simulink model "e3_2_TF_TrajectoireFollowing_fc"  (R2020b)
settings: Solver=FixedStepAuto  StartTime=0.0  StopTime=100  FixedStep=sampleTime  RelTol=1e-3  EnableMultiTasking=on
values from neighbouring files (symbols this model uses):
  saturation_psi = 2    [startSimulation.m]    (also in StartSimulation.m; start.m)
  saturation_x = 2    [startSimulation.m]    (also in StartSimulation.m; start.m)
  saturation_y = 2    [startSimulation.m]    (also in StartSimulation.m; start.m)
  saturation_z = 2    [startSimulation.m]    (also in StartSimulation.m; start.m)
libraries: simulink x11, aerolibanimutils x1

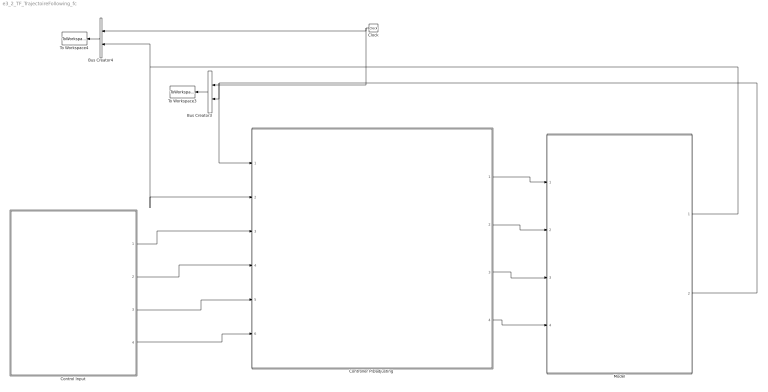
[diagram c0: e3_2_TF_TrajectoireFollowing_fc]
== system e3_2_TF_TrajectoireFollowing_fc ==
  Bus Creator3 : BusCreator  Inputs=2
  Bus Creator4 : BusCreator  Inputs=2
  Clock : Clock
  Control Input : Subsystem
  "Controller PIDadjusting " : Subsystem
  Model : Subsystem
  To Workspace3 : ToWorkspace  VariableName=r1_pos_array  SampleTime=-1
  To Workspace4 : ToWorkspace  VariableName=r1_vel_array  SampleTime=-1
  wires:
  Clock/1 -> Bus Creator4/1, Bus Creator3/1
  Bus Creator3/1 -> To Workspace3/1
  Bus Creator4/1 -> To Workspace4/1
  "Controller PIDadjusting "/1(Controller Output X) -> Model/1(Commande Input X)
  "Controller PIDadjusting "/2(Controller Output Y) -> Model/2(Commande Input Y)
  "Controller PIDadjusting "/3(Controller Output H) -> Model/3(Commande Input H)
  "Controller PIDadjusting "/4(Controller Output Psi) -> Model/4(Commande Input Psi)
  Control Input/1(ux) -> "Controller PIDadjusting "/3(Control input X)
  Control Input/2(uy) -> "Controller PIDadjusting "/4(Control input Y)
  Control Input/3(uz) -> "Controller PIDadjusting "/5(Control input H)
  Control Input/4(upsi) -> "Controller PIDadjusting "/6(Control input Psi)
  Model/2(Output Position) -> "Controller PIDadjusting "/1(Feedback Position), Bus Creator3/2
  Model/1(Output Velocity) -> "Controller PIDadjusting "/2(Feedback Velocity), Bus Creator4/2

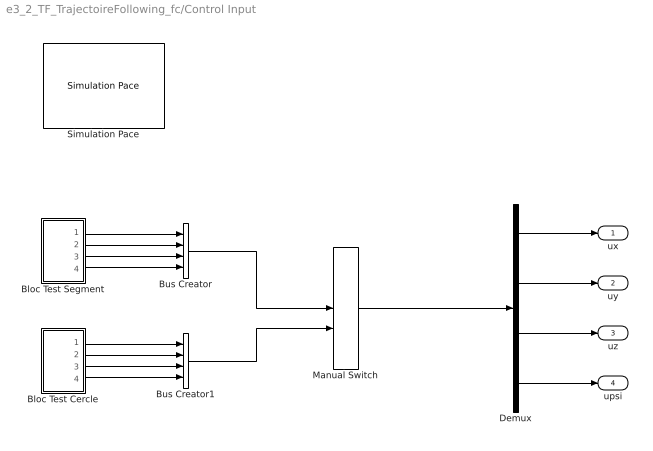
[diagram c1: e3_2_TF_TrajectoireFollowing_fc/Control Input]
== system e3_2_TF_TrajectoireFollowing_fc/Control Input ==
  Bloc Test Cercle : Subsystem
  Bloc Test Segment : Subsystem
  Bus Creator : BusCreator  Inputs=4
  Bus Creator1 : BusCreator  Inputs=4
  Demux : Demux
  Manual Switch : ManualSwitch  CurrentSetting=0
  Simulation Pace : aerolibanimutils/Simulation Pace  SimulationPace=100  SleepMode=MATLAB Thread  OutputPaceError=off  SampleTime=-1
  ux : Outport  VectorParamsAs1DForOutWhenUnconnected=off
  uy : Outport  Port=2  VectorParamsAs1DForOutWhenUnconnected=off
  uz : Outport  Port=3  VectorParamsAs1DForOutWhenUnconnected=off
  upsi : Outport  Port=4  VectorParamsAs1DForOutWhenUnconnected=off
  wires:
  Demux/2 -> uy/1
  Demux/1 -> ux/1
  Bloc Test Segment/2(uy) -> Bus Creator/2
  Demux/3 -> uz/1
  Demux/4 -> upsi/1
  Bloc Test Segment/4(upsi) -> Bus Creator/4
  Bloc Test Segment/3(uz) -> Bus Creator/3
  Bloc Test Segment/1(ux) -> Bus Creator/1
  Bus Creator/1 -> Manual Switch/1
  Bloc Test Cercle/4(upsi) -> Bus Creator1/4
  Bloc Test Cercle/3(uz) -> Bus Creator1/3
  Bloc Test Cercle/1(ux) -> Bus Creator1/1
  Bloc Test Cercle/2(uy) -> Bus Creator1/2
  Bus Creator1/1 -> Manual Switch/2
  Manual Switch/1 -> Demux/1

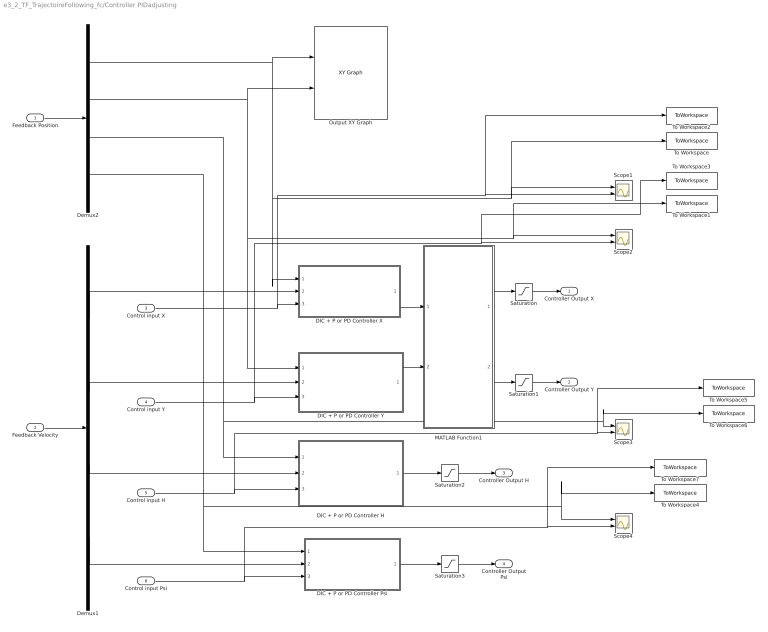
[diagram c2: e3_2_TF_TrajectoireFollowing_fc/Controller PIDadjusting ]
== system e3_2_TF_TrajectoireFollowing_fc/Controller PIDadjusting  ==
  Feedback Position : Inport
  Feedback Velocity : Inport  Port=2
  Control input X : Inport  Port=3
  Control input Y : Inport  Port=4
  Control input H : Inport  Port=5
  Control input Psi : Inport  Port=6
  DIC + P or PD Controller H : Subsystem
  DIC + P or PD Controller Psi : Subsystem
  DIC + P or PD Controller X : Subsystem
  DIC + P or PD Controller Y : Subsystem
  Demux1 : Demux
  Demux2 : Demux
  MATLAB Function1 : MATLAB Function  TreatAsAtomicUnit=on
  Output XY Graph : simulink/Sinks/XY Graph  xmin=-5  xmax=5  ymin=-5  ymax=5  st=-1
  Saturation : Saturate  UpperLimit=saturation_x  LowerLimit=-saturation_x
  Saturation1 : Saturate  UpperLimit=saturation_y  LowerLimit=-saturation_y
  Saturation2 : Saturate  UpperLimit=saturation_z  LowerLimit=-saturation_z
  Saturation3 : Saturate  UpperLimit=saturation_psi  LowerLimit=-saturation_psi
  Scope{1..4} (4 alike) : Scope  NumInputPorts=2
  To Workspace : ToWorkspace  VariableName=N4_Step2_Out_X  SampleTime=-1
  To Workspace1 : ToWorkspace  VariableName=N4_Step2_Out_Y  SampleTime=-1
  To Workspace2 : ToWorkspace  VariableName=N4_Step2_In_X  SampleTime=-1
  To Workspace3 : ToWorkspace  VariableName=N4_Step2_In_Y  SampleTime=-1
  To Workspace4 : ToWorkspace  VariableName=N4_Step2_Out_Psi  SampleTime=-1
  To Workspace5 : ToWorkspace  VariableName=N4_Step2_In_H  SampleTime=-1
  To Workspace6 : ToWorkspace  VariableName=N4_Step2_Out_H  SampleTime=-1
  To Workspace7 : ToWorkspace  VariableName=N4_Step2_In_Psi  SampleTime=-1
  Controller Output X : Outport  VectorParamsAs1DForOutWhenUnconnected=off
  Controller Output Y : Outport  Port=2  VectorParamsAs1DForOutWhenUnconnected=off
  Controller Output H : Outport  Port=3  VectorParamsAs1DForOutWhenUnconnected=off
  Controller Output Psi : Outport  Port=4  VectorParamsAs1DForOutWhenUnconnected=off
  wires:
  Feedback Position/1 -> Demux2/1
  Feedback Velocity/1 -> Demux1/1
  Demux1/2 -> DIC + P or PD Controller Y/2(Feedback Velocity Y)
  Demux2/3 -> Scope3/1, To Workspace6/1, DIC + P or PD Controller H/1(Feedback Position H)
  Demux1/1 -> DIC + P or PD Controller X/2(Feedback Velocity X)
  Demux1/3 -> DIC + P or PD Controller H/2(Feedback Velocity H)
  Control input X/1 -> To Workspace2/1, Scope1/2, DIC + P or PD Controller X/3(Control Input X)
  Control input H/1 -> Scope3/2, To Workspace5/1, DIC + P or PD Controller H/3(Control Input H)
  Saturation/1 -> Controller Output X/1
  Saturation1/1 -> Controller Output Y/1
  Saturation2/1 -> Controller Output H/1
  Saturation3/1 -> Controller Output Psi/1
  Control input Y/1 -> DIC + P or PD Controller Y/3(Control Input Y), Scope2/2, To Workspace3/1
  DIC + P or PD Controller H/1(Controller Output H) -> Saturation2/1
  DIC + P or PD Controller Psi/1(Controller Output Psi) -> Saturation3/1
  Demux2/1 -> To Workspace/1, Scope1/1, DIC + P or PD Controller X/1(Feedback Position X), Output XY Graph/1
  Demux2/2 -> DIC + P or PD Controller Y/1(Feedback Position Y), Scope2/1, To Workspace1/1, Output XY Graph/2
  Demux2/4 -> Scope4/1, To Workspace4/1, DIC + P or PD Controller Psi/1(Feedback Position Psi)
  Demux1/4 -> DIC + P or PD Controller Psi/2(Feedback Velocity Psi)
  Control input Psi/1 -> Scope4/2, To Workspace7/1, DIC + P or PD Controller Psi/3(Control input Psi)
  DIC + P or PD Controller Y/1(Controller Output Y) -> MATLAB Function1/2(eay)
  MATLAB Function1/2(phi) -> Saturation1/1
  MATLAB Function1/1(theta) -> Saturation/1
  DIC + P or PD Controller X/1(Controller Output X) -> MATLAB Function1/1(eax)

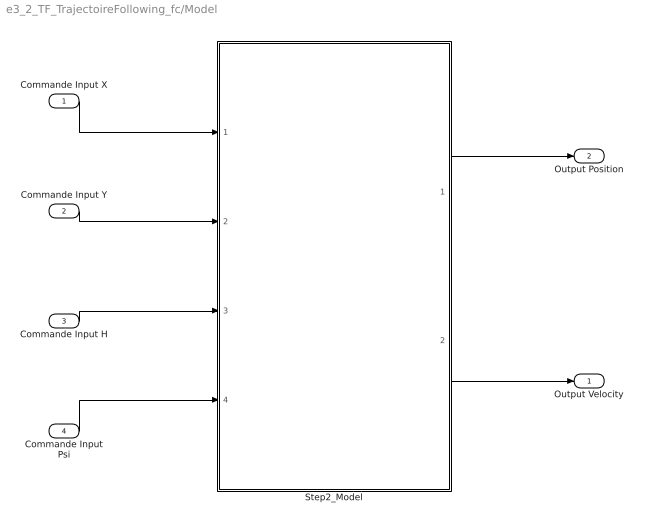
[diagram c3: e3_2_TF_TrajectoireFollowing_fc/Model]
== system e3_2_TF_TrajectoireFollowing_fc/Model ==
  Commande Input X : Inport
  Commande Input Y : Inport  Port=2
  Commande Input H : Inport  Port=3
  Commande Input Psi : Inport  Port=4
  Step2_Model : Subsystem
  Output Velocity : Outport  VectorParamsAs1DForOutWhenUnconnected=off
  Output Position : Outport  Port=2  VectorParamsAs1DForOutWhenUnconnected=off
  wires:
  Commande Input Y/1 -> Step2_Model/2(In2)
  Commande Input Psi/1 -> Step2_Model/4(In4)
  Commande Input H/1 -> Step2_Model/3(In3)
  Step2_Model/1(Position) -> Output Position/1
  Commande Input X/1 -> Step2_Model/1(In1)
  Step2_Model/2(Velocity) -> Output Velocity/1

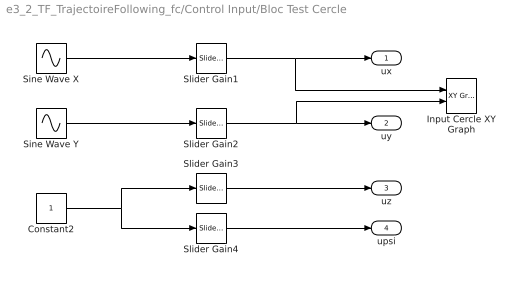
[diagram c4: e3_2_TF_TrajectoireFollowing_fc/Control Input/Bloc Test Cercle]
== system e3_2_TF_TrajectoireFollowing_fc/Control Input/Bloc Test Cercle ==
  Constant2 : Constant
  Input Cercle XY Graph : simulink/Sinks/XY Graph  Commented=on  xmin=-2  xmax=2  ymin=-2  ymax=2  st=-1
  Sine Wave X : Sin  Frequency=0.65  SampleTime=0
  Sine Wave Y : Sin  Frequency=0.65  Phase=pi/2  SampleTime=0
  Slider Gain1 : simulink/Math Operations/Slider Gain  gain=1  low=-10  high=10
  Slider Gain2 : simulink/Math Operations/Slider Gain  gain=1  low=-10  high=10
  Slider Gain3 : simulink/Math Operations/Slider Gain  gain=1  low=-3  high=3
  Slider Gain4 : simulink/Math Operations/Slider Gain  gain=0  low=-2  high=2
  ux : Outport  VectorParamsAs1DForOutWhenUnconnected=off
  uy : Outport  Port=2  VectorParamsAs1DForOutWhenUnconnected=off
  uz : Outport  Port=3  VectorParamsAs1DForOutWhenUnconnected=off
  upsi : Outport  Port=4  VectorParamsAs1DForOutWhenUnconnected=off
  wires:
  Slider Gain2/1 -> Input Cercle XY Graph/2, uy/1
  Slider Gain3/1 -> uz/1
  Slider Gain4/1 -> upsi/1
  Slider Gain1/1 -> Input Cercle XY Graph/1, ux/1
  Constant2/1 -> Slider Gain4/1, Slider Gain3/1
  Sine Wave Y/1 -> Slider Gain2/1
  Sine Wave X/1 -> Slider Gain1/1

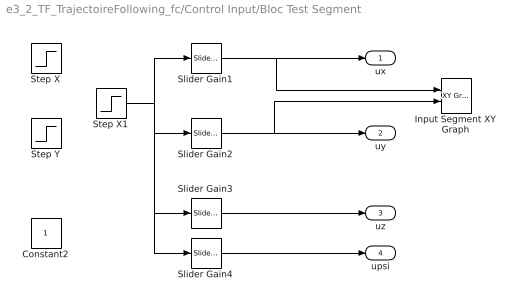
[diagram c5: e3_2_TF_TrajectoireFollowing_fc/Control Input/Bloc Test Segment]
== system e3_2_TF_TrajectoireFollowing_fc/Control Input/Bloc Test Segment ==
  Constant2 : Constant
  Input Segment XY Graph : simulink/Sinks/XY Graph  Commented=on  xmin=-2  xmax=2  ymin=-2  ymax=2  st=-1
  Slider Gain1 : simulink/Math Operations/Slider Gain  gain=1  low=-10  high=10
  Slider Gain2 : simulink/Math Operations/Slider Gain  gain=0  low=-10  high=10
  Slider Gain3 : simulink/Math Operations/Slider Gain  gain=0  low=-2  high=2
  Slider Gain4 : simulink/Math Operations/Slider Gain  gain=0  low=-2  high=2
  Step X : Step  SampleTime=0
  Step X1 : Step  Time=5  SampleTime=0
  Step Y : Step  After=-1  SampleTime=0
  ux : Outport  VectorParamsAs1DForOutWhenUnconnected=off
  uy : Outport  Port=2  VectorParamsAs1DForOutWhenUnconnected=off
  uz : Outport  Port=3  VectorParamsAs1DForOutWhenUnconnected=off
  upsi : Outport  Port=4  VectorParamsAs1DForOutWhenUnconnected=off
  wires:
  Constant2/1 -> ?
  Slider Gain1/1 -> Input Segment XY Graph/1, ux/1
  Slider Gain2/1 -> Input Segment XY Graph/2, uy/1
  Slider Gain3/1 -> uz/1
  Slider Gain4/1 -> upsi/1
  Step X1/1 -> Slider Gain1/1, Slider Gain2/1, Slider Gain3/1, Slider Gain4/1

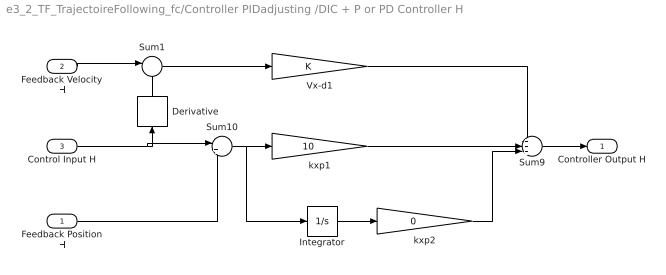
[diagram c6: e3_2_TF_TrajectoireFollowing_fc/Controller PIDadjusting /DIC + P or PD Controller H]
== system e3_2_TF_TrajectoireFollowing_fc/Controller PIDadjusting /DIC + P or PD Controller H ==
  Feedback Position H : Inport
  Feedback Velocity H : Inport  Port=2
  Control Input H : Inport  Port=3
  Derivative : Derivative
  Integrator : Integrator
  Sum1 : Sum  Inputs=|-+
  Sum10 : Sum  Inputs=|+-
  Sum9 : Sum  Inputs=+++|
  Vx-d1 : Gain
  kxp1 : Gain  Gain=10
  kxp2 : Gain  Gain=0
  Controller Output H : Outport  VectorParamsAs1DForOutWhenUnconnected=off
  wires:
  Sum9/1 -> Controller Output H/1
  Sum10/1 -> Integrator/1, kxp1/1
  kxp1/1 -> Sum9/2
  Vx-d1/1 -> Sum9/1
  Feedback Velocity H/1 -> Sum1/1
  Sum1/1 -> Vx-d1/1
  Integrator/1 -> kxp2/1
  kxp2/1 -> Sum9/3
  Control Input H/1 -> Sum10/1, Derivative/1
  Feedback Position H/1 -> Sum10/2
  Derivative/1 -> Sum1/2

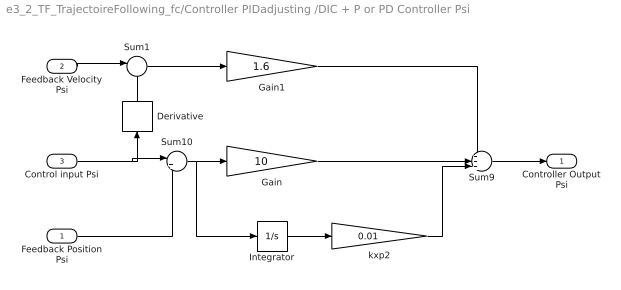
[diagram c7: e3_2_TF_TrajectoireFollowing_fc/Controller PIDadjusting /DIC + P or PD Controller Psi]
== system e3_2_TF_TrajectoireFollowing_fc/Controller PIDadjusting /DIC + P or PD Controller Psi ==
  Feedback Position Psi : Inport
  Feedback Velocity Psi : Inport  Port=2
  Control input Psi : Inport  Port=3
  Derivative : Derivative
  Gain : Gain  Gain=10
  Gain1 : Gain  Gain=1.6
  Integrator : Integrator
  Sum1 : Sum  Inputs=|-+
  Sum10 : Sum  Inputs=|+-
  Sum9 : Sum  Inputs=+++|
  kxp2 : Gain  Gain=0.01
  Controller Output Psi : Outport  VectorParamsAs1DForOutWhenUnconnected=off
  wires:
  Sum9/1 -> Controller Output Psi/1
  kxp2/1 -> Sum9/3
  Control input Psi/1 -> Sum10/1, Derivative/1
  Gain1/1 -> Sum9/1
  Sum10/1 -> Gain/1, Integrator/1
  Integrator/1 -> kxp2/1
  Feedback Velocity Psi/1 -> Sum1/1
  Sum1/1 -> Gain1/1
  Gain/1 -> Sum9/2
  Derivative/1 -> Sum1/2
  Feedback Position Psi/1 -> Sum10/2

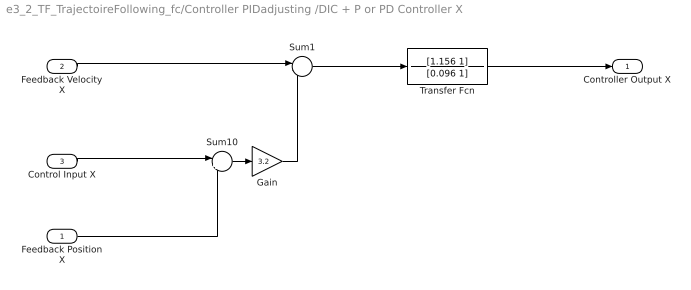
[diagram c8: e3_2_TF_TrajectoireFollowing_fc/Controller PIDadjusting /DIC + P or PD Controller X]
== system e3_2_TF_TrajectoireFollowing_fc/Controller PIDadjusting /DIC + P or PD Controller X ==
  Feedback Position X : Inport
  Feedback Velocity X : Inport  Port=2
  Control Input X : Inport  Port=3
  Gain : Gain  Gain=3.2
  Sum1 : Sum  Inputs=|-+
  Sum10 : Sum  Inputs=|+-
  Transfer Fcn : TransferFcn  Numerator=[1.156 1]  Denominator=[0.096 1]
  Controller Output X : Outport  VectorParamsAs1DForOutWhenUnconnected=off
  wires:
  Feedback Velocity X/1 -> Sum1/1
  Feedback Position X/1 -> Sum10/2
  Control Input X/1 -> Sum10/1
  Sum1/1 -> Transfer Fcn/1
  Sum10/1 -> Gain/1
  Transfer Fcn/1 -> Controller Output X/1
  Gain/1 -> Sum1/2

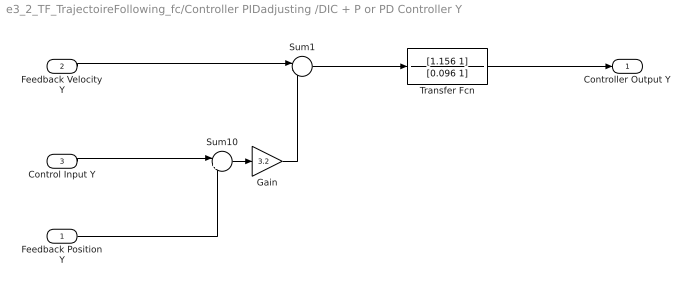
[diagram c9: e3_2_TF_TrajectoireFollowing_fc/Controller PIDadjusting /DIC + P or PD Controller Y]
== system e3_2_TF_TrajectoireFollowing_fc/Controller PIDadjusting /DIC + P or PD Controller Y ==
  Feedback Position Y : Inport
  Feedback Velocity Y : Inport  Port=2
  Control Input Y : Inport  Port=3
  Gain : Gain  Gain=3.2
  Sum1 : Sum  Inputs=|-+
  Sum10 : Sum  Inputs=|+-
  Transfer Fcn : TransferFcn  Numerator=[1.156 1]  Denominator=[0.096 1]
  Controller Output Y : Outport  VectorParamsAs1DForOutWhenUnconnected=off
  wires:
  Sum1/1 -> Transfer Fcn/1
  Sum10/1 -> Gain/1
  Feedback Position Y/1 -> Sum10/2
  Gain/1 -> Sum1/2
  Control Input Y/1 -> Sum10/1
  Feedback Velocity Y/1 -> Sum1/1
  Transfer Fcn/1 -> Controller Output Y/1

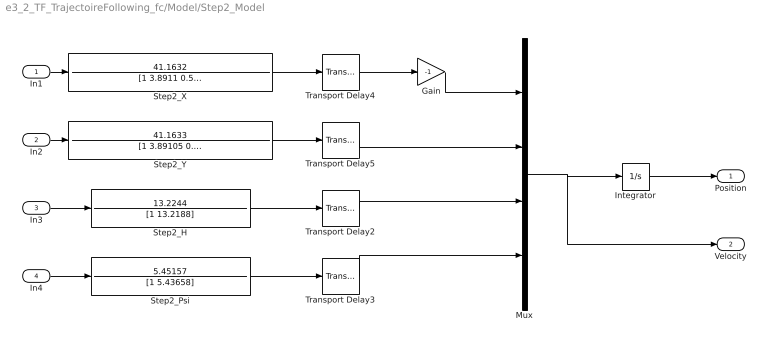
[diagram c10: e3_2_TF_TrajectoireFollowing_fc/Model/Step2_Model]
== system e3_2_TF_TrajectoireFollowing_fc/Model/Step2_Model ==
  In1 : Inport
  In2 : Inport  Port=2
  In3 : Inport  Port=3
  In4 : Inport  Port=4
  Gain : Gain  Gain=-1
  Integrator : Integrator
  Mux : Mux
  Step2_H : TransferFcn  Numerator=13.2244  Denominator=[1 13.2188]
  Step2_Psi : TransferFcn  Numerator=5.45157  Denominator=[1 5.43658]
  Step2_X : TransferFcn  Numerator=41.1632  Denominator=[1 3.8911 0.529635]
  Step2_Y : TransferFcn  Numerator=41.1633  Denominator=[1 3.89105 0.529839]
  Transport Delay2 : TransportDelay  DelayTime=0.0344
  Transport Delay3 : TransportDelay  DelayTime=0.0313
  Transport Delay4 : TransportDelay  DelayTime=0.0289
  Transport Delay5 : TransportDelay  DelayTime=0.0289
  Position : Outport  VectorParamsAs1DForOutWhenUnconnected=off
  Velocity : Outport  Port=2  VectorParamsAs1DForOutWhenUnconnected=off
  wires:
  Transport Delay2/1 -> Mux/3
  In2/1 -> Step2_Y/1
  In4/1 -> Step2_Psi/1
  Transport Delay3/1 -> Mux/4
  In1/1 -> Step2_X/1
  In3/1 -> Step2_H/1
  Step2_H/1 -> Transport Delay2/1
  Step2_Y/1 -> Transport Delay5/1
  Step2_X/1 -> Transport Delay4/1
  Step2_Psi/1 -> Transport Delay3/1
  Transport Delay4/1 -> Gain/1
  Transport Delay5/1 -> Mux/2
  Integrator/1 -> Position/1
  Mux/1 -> Velocity/1, Integrator/1
  Gain/1 -> Mux/1

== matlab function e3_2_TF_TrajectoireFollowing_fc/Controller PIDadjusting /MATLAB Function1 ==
function [theta,phi] = fcn(eax,eay)
g=9.8;

theta =-eax/g;% vx
phi =eay/g;% vy
